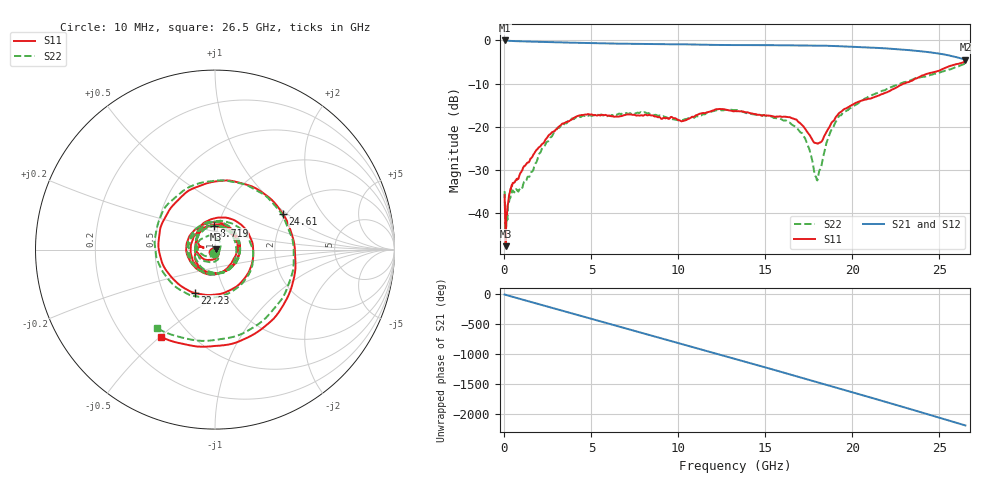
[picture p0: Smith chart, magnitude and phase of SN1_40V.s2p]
!Agilent Technologies,N5222A,MY51421700,A.10.00.00
!Agilent N5222A: A.10.00.00
!Date: Thursday, April 02, 2015 22:41:07
!Correction: S11(Full 2 Port(1,2))
!S21(Full 2 Port(1,2))
!S12(Full 2 Port(1,2))
!S22(Full 2 Port(1,2))
!S2P File: Measurements: S11, S21, S12, S22:
# Hz S  dB  R 50
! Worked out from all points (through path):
!   801 points, 10 MHz to 26.5 GHz, reference 50 ohm
!   highest |S21| = 0.01 dB at 10 MHz (marker M1); lowest = -4.4 dB at 26.5 GHz (marker M2)
!   group delay of S21, straight-line fit = 228 ps
!   lowest |S11| = -47.6 dB at 76.22 MHz (marker M3), VSWR 1.01, Z = 50.3 + j0.258 ohm
!   |S11| at or under -10 dB: start of sweep to 22.94 GHz
!   |S22| runs from -47.4 to -5.3 dB; largest |S21 - S12| = 0.0025
!   S11 on the Smith chart (normalised r, x): 10 MHz: 0.98, -0.03; 8.719 GHz: 0.95, +0.26; 22.23 GHz: 0.71, -0.37; 24.61 GHz: 1.92, +0.93; 26.5 GHz: 0.35, -0.51
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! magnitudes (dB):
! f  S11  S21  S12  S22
! 10 MHz  -35.8  0.0  0.0  -34.8
! 76.22 MHz  -47.6  0.0  0.0  -47.4
! 175.6 MHz  -38.2  -0.1  -0.1  -41.5
! 473.6 MHz  -33.0  -0.1  -0.1  -34.7
! 937.1 MHz  -30.5  -0.2  -0.2  -34.3
! 1.864 GHz  -25.2  -0.3  -0.3  -27.9
! 3.123 GHz  -20.0  -0.4  -0.4  -20.2
! 4.447 GHz  -17.2  -0.6  -0.6  -17.5
! 8.719 GHz  -17.5  -0.8  -0.8  -17.2
! 8.851 GHz  -17.8  -0.8  -0.8  -17.4
! 10.11 GHz  -18.5  -0.9  -0.9  -18.5
! 13.26 GHz  -16.3  -1.1  -1.1  -16.1
! 16.53 GHz  -18.0  -1.1  -1.1  -19.5
! 17.23 GHz  -20.1  -1.1  -1.1  -22.3
! 17.69 GHz  -22.9  -1.2  -1.2  -27.7
! 17.99 GHz  -23.8  -1.2  -1.2  -32.4
! 18.62 GHz  -20.4  -1.2  -1.2  -22.5
! 19.18 GHz  -17.1  -1.3  -1.3  -17.9
! 22.1 GHz  -11.8  -1.9  -1.9  -11.1
! 22.23 GHz  -11.5  -1.9  -1.9  -10.8
! 24.61 GHz  -7.4  -2.8  -2.8  -7.9
! 26.5 GHz  -4.9  -4.4  -4.4  -5.3
